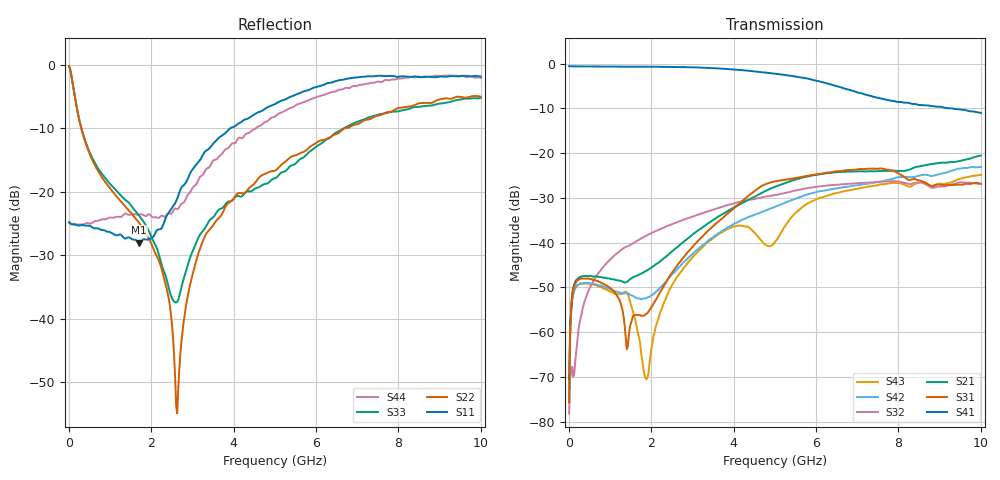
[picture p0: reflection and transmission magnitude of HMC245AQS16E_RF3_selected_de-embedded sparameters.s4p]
! Device:	HMC245AQS16E
! Description:	GaAs MMIC SP3T Non-Reflective Switch
! Package:	LP3E - 16 pin 3x3mm QFN plastic package
! Frequency:	DC -  3.5 GHz
! Ports:
! RFC = Port 1
! RF1 = Port 2
! RF2 = Port 3
! RF3 = Port 4
! State: RF3 Selected
! Supply Voltage:
! Vdd = 5 V
! Control Voltages:
! VA  = 0 V
! VB  = 5 V
! Data:	Data was collected using a calibrated network analyzer with AFR software.
!	Fixtures were calculated using AFR and fixturing was applied to collect
!	this Deembedded  S Parameter data of HMC245AQS16E
! Note:	Analog Devices supplies this data as a sample of measured data at the package pin
!	for this product.  Your particular data for this product may vary.
!	Data was taken at 25 degrees C.
!	Analog Devices reserves the right to change this data at anytime.
# GHz S  dB  R 50
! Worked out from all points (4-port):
!   401 points, 10 MHz to 10 GHz, reference 50 ohm
!   strongest paths, dB at 10 MHz, 2.507 GHz, 5.005 GHz, 7.503 GHz, 10 GHz:
!     S41: -0.6, -0.7, -2.2, -7.7, -11.0
!     S31: -75.8, -46.7, -26.3, -23.5, -26.9
!     S21: -75.6, -41.9, -27.5, -24.0, -20.5
!     S32: -78.2, -35.9, -29.4, -26.5, -26.9
!     S42: -73.6, -47.1, -32.0, -26.5, -23.1
!     S43: -70.5, -49.5, -39.8, -27.1, -24.9
!   lowest |S11| = -28.0 dB at 1.708 GHz (marker M1), VSWR 1.08, Z = 51.4 - j3.79 ohm
!   |S11| at or under -10 dB: start of sweep to 3.914 GHz
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0.01  -24.84 -0.7  -67.91 109.2  -75.09 83.8  -0.58 -0.4
      -75.59 76.6  -0.18 -5.8  -77.95 142.7  -79.00 55.5
      -75.80 73.8  -78.16 27.0  -0.18 -5.7  -69.64 95.7
      -0.57 -0.4  -73.57 78.0  -70.51 49.9  -24.67 -0.4
0.2098  -25.28 -7.1  -48.17 33.8  -48.46 28.4  -0.63 -6.6
        -48.16 33.1  -7.27 -60.3  -61.76 110.6  -49.46 22.4
        -48.51 28.6  -61.89 110.6  -7.19 -60.2  -49.64 26.1
        -0.63 -6.6  -49.42 22.1  -49.59 26.2  -25.15 -3.9
1.7083  -27.98 -67.2  -47.14 55.5  -56.35 50.1  -0.69 -53.0
        -47.13 55.4  -24.88 -63.8  -39.35 86.3  -52.61 -103.6
        -56.20 50.0  -39.33 86.3  -23.72 -68.4  -61.53 -72.5
        -0.69 -53.0  -52.49 -103.5  -61.31 -70.3  -23.53 -39.1
2.632375  -21.06 -162.8  -41.03 78.3  -45.12 107.5  -0.74 -83.2
          -41.06 78.3  -54.90 55.8  -35.43 77.4  -45.97 161.3
          -45.11 107.3  -35.41 77.4  -37.32 -157.0  -47.61 116.0
          -0.75 -83.2  -45.99 161.4  -47.62 116.5  -22.71 -111.4
4.080925  -9.39 131.9  -31.77 63.3  -31.72 79.3  -1.38 -133.0
          -31.78 63.3  -20.36 102.9  -31.04 57.0  -35.51 90.3
          -31.72 79.4  -31.03 56.9  -20.63 127.5  -36.25 50.4
          -1.38 -133.0  -35.50 90.2  -36.26 50.3  -11.87 150.5
6.428575  -2.65 53.2  -24.32 2.3  -24.16 -15.5  -4.84 146.8
          -24.32 2.4  -11.02 55.0  -27.09 24.9  -27.96 1.6
          -24.17 -15.5  -27.10 24.9  -10.91 63.4  -29.06 13.5
          -4.84 146.9  -27.97 1.7  -29.06 13.5  -4.21 58.2
10  -1.82 -27.6  -20.55 -68.6  -26.88 -115.2  -11.03 54.9
    -20.55 -68.6  -5.01 -9.1  -26.86 -51.8  -23.09 -124.2
    -26.87 -115.5  -26.90 -51.7  -5.18 -0.9  -24.86 -102.9
    -11.04 54.9  -23.08 -124.1  -24.85 -102.7  -2.04 -25.4
